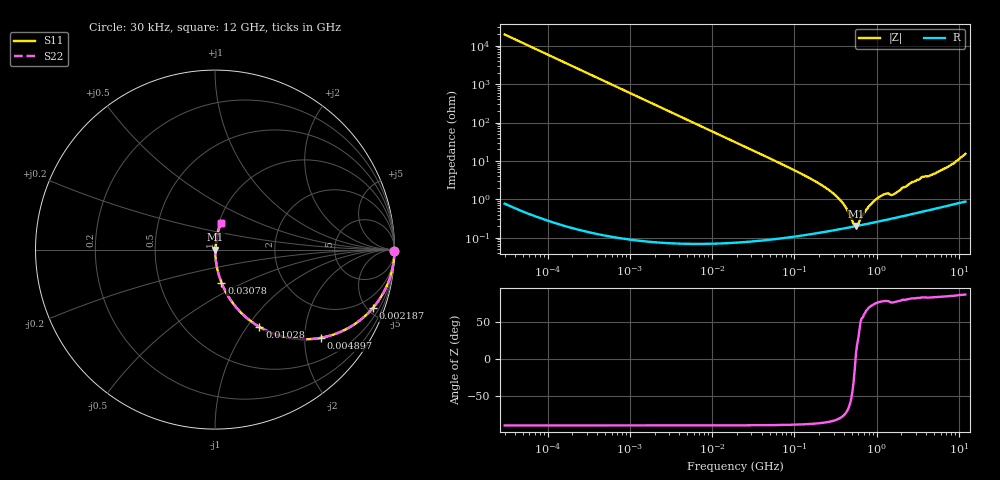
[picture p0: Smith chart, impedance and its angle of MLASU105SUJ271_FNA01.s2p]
! MLASU105SUJ271_FNA01  S-PARAMETER MODEL  ( General Type )
! Model Generated by TAIYO YUDEN Corporation (http://www.ty-top.com)
! Version 3.0
! TAIYO YUDEN Control No. 120810
! Copyright(c) 2003 TAIYO YUDEN CO.,LTD. All Rights Reserved.
! Product Description (link to TY-COMPAS)
! https://ds.yuden.co.jp/TYCOMPAS/or/detail?pn=MLASU105SUJ271JFNA01&u=M
! Products Name : Multilayer Ceramic Capacitors
! Characteristics :
!  Capacitance : 270 pF , Rated Voltage : 50V , TCC : UJ / U2J
!  Case Size : 1.0 x 0.5 / 0.039 x 0.02 [mm/inch] , Thickness : 0.5 / 0.02 [mm/inch]
!  (Conditions: Temperature = 25 degC , DC Bias Current/Voltage = 0A / 0V)
! External Node Assignments :
!  1  o---| |---o  2
! GND o---------o GND
! Frequency Range : 0.03MHz  -  12000MHz  [ 401 STEP ]
# MHz S RI R 50
! Freq[MHz].  S11 Real  S11 Imag  S21 Real  S21 Imag  S12 Real  S12 Imag  S22 Real  S22 Imag
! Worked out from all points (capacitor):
!   401 points, 30 kHz to 12 GHz, reference 50 ohm
!   read as one part in series: C = 270 pF near 32 kHz
!   lowest |Z| = 201 mohm at 560.7 MHz (marker M1)
!   series resonance near 554.6 MHz, so ESL is about 310 pH
!   S11 on the Smith chart (normalised r, x): 30 kHz: open; 2.187 MHz: 1.00, -5.39; 4.897 MHz: 1.00, -2.41; 10.28 MHz: 1.00, -1.15; 30.78 MHz: 1.00, -0.38; 12 GHz: 1.02, +0.31
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0.03  1 -0.00509  2.61e-05 0.00509  2.61e-05 0.00509  1 -0.00509
0.260295  0.9981 -0.0441  0.00195 0.0441  0.00195 0.0441  0.9981 -0.0441
0.831097  0.9805 -0.1382  0.0195 0.1382  0.0195 0.1382  0.9805 -0.1382
2.186786  0.879 -0.326  0.121 0.326  0.121 0.326  0.879 -0.326
2.258455  0.8719 -0.334  0.1281 0.334  0.1281 0.334  0.8719 -0.334
4.897055  0.5916 -0.4913  0.4084 0.4913  0.4084 0.4913  0.5916 -0.4913
10.28143  0.2475 -0.431  0.7525 0.431  0.7525 0.431  0.2475 -0.431
18.97367  0.0884 -0.2827  0.9116 0.2827  0.9116 0.2827  0.0884 -0.2827
30.77716  0.0359 -0.1839  0.9641 0.1839  0.9641 0.1839  0.0359 -0.1839
164.6252  0.00231 -0.0325  0.9977 0.0325  0.9977 0.0325  0.00231 -0.0325
345.6326  0.00175 -0.0104  0.9983 0.0104  0.9983 0.0104  0.00175 -0.0104
419.4166  0.00181 -0.006  0.9982 0.006  0.9982 0.006  0.00181 -0.006
525.6319  0.00194 -0.00114  0.9981 0.00114  0.9981 0.00114  0.00194 -0.00114
560.6502  0.002 0.000239  0.998 -0.000239  0.998 -0.000239  0.002 0.000239
774.0045  0.00232 0.00528  0.9977 -0.00528  0.9977 -0.00528  0.00232 0.00528
939.2353  0.00257 0.00866  0.9974 -0.00866  0.9974 -0.00866  0.00257 0.00866
1215.67  0.00298 0.0129  0.997 -0.0129  0.997 -0.0129  0.00298 0.0129
1428.372  0.0032 0.0134  0.9968 -0.0134  0.9968 -0.0134  0.0032 0.0134
1625.032  0.00339 0.0132  0.9966 -0.0132  0.9966 -0.0132  0.00339 0.0132
2722.352  0.00488 0.0276  0.9951 -0.0276  0.9951 -0.0276  0.00488 0.0276
7397.824  0.0115 0.0686  0.9885 -0.0686  0.9885 -0.0686  0.0115 0.0686
12000  0.0309 0.1469  0.9691 -0.1469  0.9691 -0.1469  0.0309 0.1469
